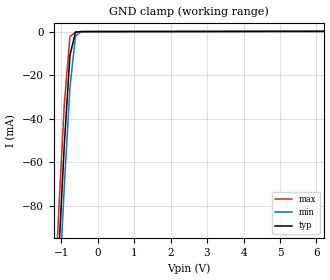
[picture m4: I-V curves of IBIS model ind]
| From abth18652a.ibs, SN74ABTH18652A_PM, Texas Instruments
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[Model]   ind
| input buffer with pulldown resistor
| ind.abh (95186 ALEY)
| pad.abh (95272 ALEY)
Model_type   Input
Polarity   Non-Inverting
| Signals   OE
Vinl = 0.8V
Vinh = 2.0V
| variable   typ   min   max
C_comp   5pF   NA   NA
| variable   typ   min   max
[Voltage range]   5.0V   4.5V   5.5V
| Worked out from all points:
|   GND clamp passes 1 mA (typ) near -0.62 V on its own axis
[gnd_clamp]
|   50C:5V:   100C:4.5V:weak   0C:5.5V:strong
|   Voltage   I(typ)   I(min)   I(max)
-5V       -1.557A    -1.574A    -1.54A
-1.212V   -153.4mA   -173.2mA   -133.8mA
-1.061V   -100.8mA   -120.6mA   -81.22mA
-909.1mV  -50.98mA   -70.19mA   -32.51mA
-757.6mV  -10.86mA   -25.7mA    -2.27mA
-606.1mV  -236.1uA   -2.11mA    -257.2uA
-454.5mV  -7.748uA   -37.81uA   -25.63uA
-303mV    -4.485uA   -3.326uA   -7.127uA
10V       148.2uA    98.84uA    237.2uA
